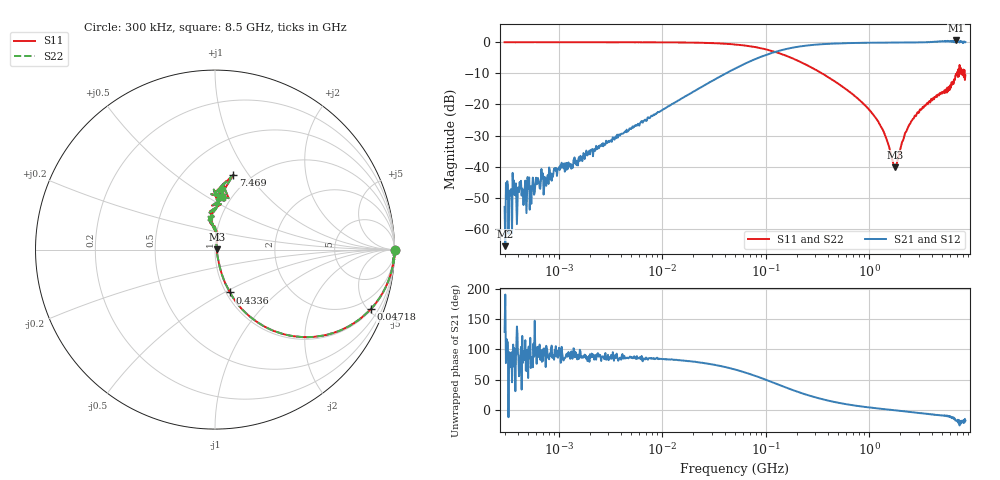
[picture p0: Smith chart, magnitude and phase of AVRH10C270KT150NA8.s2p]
! S-Parameter Data Generated by TDK Corporation
! Copyright(C) 2023 TDK Corporation.
! All Rights Reserved.
! TDK P/N: AVRH10C270KT150NA8 (Varistor)
! Property: V1mA=27V
! Size(LxWxT): 1x0.5x0.5mm
! Model Type: s2p (Touchstone File Format Version 1.0)
! Frequency: DC=Yes Start=0.3MHz Stop=8500MHz 802points Log-sweep
! Model Generated on Oct. 12, 2023
! Port Assignments:
!  1 ---N--- 2
! Applicable Conditions:
!  Temperature = 25 degC
!  DC Bias Voltage = 0 V
!  Small Signal Operation
! Terms and conditions regarding TDK Simulation Models
! (1)This simulation model is being provided solely for informational purposes. Please refer to the specifications of the products in terms of detailed characteristics of such products.
! (2)In no event shall TDK Corporation of any of its subsidiaries be liable for any loss or damage arising, directly or indirectly,
!  From any information contained in this simulation model, including, but not limited to loss or damages arising from any inaccuracies, omissions or errors in connection with such information.
! (3)Any and all copyrights on this simulation model are owned by TDK Corporation.
!  Duplication or redistribution of this simulation model without prior written permission from TDK Corporation is prohibited.
! (4)This simulation model is subject to any modification or change without any prior notice.
! (5)Neither TDK Corporation nor any of its subsidiaries shall make any warranty, express or implied,
!  Including but not limited to the correctness, implied warranties of merchantability and fitness for a particular purpose with respect to this simulation models.
! (6)The use of this simulation model shall be deemed to have consented to the terms and conditions hereof.
# Hz S MA R 50
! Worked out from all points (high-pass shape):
!   801 points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, 300 kHz to 8.5 GHz, reference 50 ohm
!   highest |S21| = 0.56 dB at 6.906 GHz (marker M1); lowest = -65.6 dB at 304.5 kHz (marker M2)
!   |S21| within 3 dB of the highest: 146.7 MHz to end of sweep
!   lowest |S11| = -40.2 dB at 1.787 GHz (marker M3), VSWR 1.02, Z = 51 + j0.145 ohm
!   |S11| at or under -10 dB: 349.2 MHz to 7.049 GHz (6.7 GHz wide, 181 % of centre); 7.875 GHz to 8.06 GHz (185.6 MHz wide, 2.33 % of centre); 8.344 GHz to end of sweep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
!   |S22| runs from -40.2 to 0.0 dB; largest |S21 - S12| = 0
!   S11 on the Smith chart (normalised r, x): 300 kHz: open; 47.18 MHz: 1.08, -5.23; 433.6 MHz: 1.04, -0.53; 7.469 GHz: 0.83, +0.85; 8.5 GHz: 0.90, +0.58
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300000  1.001 -0.1  0.002258 129.0  0.002258 129.0  1.001 -0.1
304501  1.001 0.0  0.0005276 -169.8  0.0005276 -169.8  1.001 0.0
327007  0.9992 0.0  0.0008357 -11.5  0.0008357 -11.5  0.9992 0.0
336009  0.9986 -0.2  0.004109 70.4  0.004109 70.4  0.9986 -0.2
349513  1 -0.2  0.0028 95.4  0.0028 95.4  1 -0.2
390024  1.001 -0.1  0.002415 111.6  0.002415 111.6  1.001 -0.1
425693  0.9996 -0.3  0.004508 85.2  0.004508 85.2  0.9996 -0.3
469099  0.9995 -0.2  0.004352 82.7  0.004352 82.7  0.9995 -0.2
1667335  1 -0.8  0.01391 89.4  0.01391 89.4  1 -0.8
9160262  0.995 -4.3  0.07585 84.0  0.07585 84.0  0.995 -4.3
4.717537e7  0.9292 -20.8  0.3551 68.3  0.3551 68.3  0.9292 -20.8
5.049752e7  0.921 -22.1  0.3764 67.1  0.3764 67.1  0.921 -22.1
1.218347e8  0.7031 -43.9  0.6938 44.7  0.6938 44.7  0.7031 -43.9
2.804659e8  0.3881 -64.3  0.9025 22.8  0.9025 22.8  0.3881 -64.3
4.335956e8  0.2528 -70.7  0.9468 14.6  0.9468 14.6  0.2528 -70.7
1.010223e9  0.08066 -74.3  0.9812 4.5  0.9812 4.5  0.08066 -74.3
1.542892e9  0.02199 -57.6  0.9884 1.1  0.9884 1.1  0.02199 -57.6
1.787118e9  0.009808 8.3  0.9903 -0.1  0.9903 -0.1  0.009808 8.3
2.641315e9  0.05838 78.7  0.9902 -3.3  0.9902 -3.3  0.05838 78.7
6.905944e9  0.3098 94.0  1.067 -16.8  1.067 -16.8  0.3098 94.0
7.468552e9  0.4299 76.2  0.9896 -25.0  0.9896 -25.0  0.4299 76.2
8.5e9  0.2935 82.7  1.006 -16.8  1.006 -16.8  0.2935 82.7
